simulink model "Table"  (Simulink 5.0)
settings: Solver=FixedStepDiscrete  SolverMode=SingleTasking  StartTime=0.0  StopTime=inf  FixedStep=samplePeriod  RelTol=1e-3  AbsTol=1e-6
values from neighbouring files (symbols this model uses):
  a0 = zeros(1, nAct)    [initialize.m]    (also in quake.m = 0; rspect.m = 1)
  actParamsX = [bulkModulus	* pressCanon,    [initialize.m]
  actParamsY = [bulkModulus	* pressCanon,    [initialize.m]
  actParamsZ = [bulkModulus	* pressCanon,    [initialize.m]
  azMask = zeros(nAcc, 1)    [initialize.m]
  bal = [[ 1  1  1  1  0  0  0  0  0  0  0  0]    [initialize.m]
  cmap = jet    [initialize.m]    (also in tableAnimation.m = self.cmap)
  ea_t = zeros(3, nAcc)    [initialize.m]
  faces = nAct               			+ [ 1  2  3  4    [initialize.m]    (also in tableAnimation.m = self.faces)
  flowCanon = 63090.2    [initialize.m]
  fmax = zeros(nAct, 1)    [initialize.m]
  gasConstant = 1.8    [initialize.m]
  gee = 1.0    (= 1)    [initialize.m]    (also in accelA2T.m = h(24); accelT2A.m = h(24); Test.m)
  inertia = [Ixx 0 0; 0 Iyy 0; 0 0 Izz]    [initialize.m]
  inertiaCanon = 0.1130    (= 0.113)    [initialize.m]
  linAccelCanon = 9800.0    (= 9800)    [initialize.m]    (also in accelA2T.m = h(19); accelT2A.m = h(19); Test.m)
  lines = nAct               			+ [ 1  2  3  4  1    				5  6  7  8  5    				9 10 11 12  9    				0  2  6 10       				0  3  7 11       				0  4  8 12  0];  	lines(find(lines==nAct)) = 0    [initialize.m]    (also in tableAnimation.m = self.lines; viewer.m = 1)
  linVelocCanon = 1000.0    (= 1000)    [initialize.m]    (also in Test.m)
  mass = [massX massY massZ]'    [initialize.m]
  massCanon = 0.4535924e-06    (= 4.535924e-07)    [initialize.m]
  maxDispl = [maxDisplX  			maxDisplY  			maxDisplZ  			maxDisplZ * linVelocCanon / rollRadius  * 180/pi  			maxDisplZ * linVelocCanon / pitchRadius * 180/pi  			min(maxDisplX, maxDisplY) * linVelocCanon / yawRadius * 180/pi]    [initialize.m]
  maxOilVolume = volume * (1 - (precharge/supplyPress)^(1/gasConstant))    (= 32.2704137442)    [initialize.m]
  maxVeloc = [maxVelocX  			maxVelocY  			maxVelocZ  			maxVelocZ * linVelocCanon / rollRadius  * 180/pi  			maxVelocZ * linVelocCanon / pitchRadius * 180/pi  			min(maxVelocX, maxVelocY) * linVelocCanon / yawRadius * 180/pi]    [initialize.m]
  minDispl = -maxDispl    [initialize.m]
  minVeloc = -maxVeloc    [initialize.m]
  nAct = size(rt_t, 2)    [initialize.m]    (also in tableAnimation.m = self.nAct)
  precharge = 2000    [initialize.m]
  pumpFlow = 1e10    (= 10000000000)    [initialize.m]
  ra_t = [  -20.0   -20.0   -92.0 -2590.0  2590.0   -62.0 -2133.0 -2133.0  2133.0  2133.0   -62.0    [initialize.m]    (also in accelA2T.m = [-h9   -h9 -h15 -h10  h10 -h14 -h12 -h12  h12  h12 -h16; accelT2A.m = [-h9   -h9 -h15 -h10  h10 -h14 -h12 -h12  h12  h12 -h16)
  rb_w = [-5692.1 -5692.1  5692.1  5692.1 -2500.0 -2500.0  2500.0  2500.0 -2400.0 -2400.0  2400.0  2400.0    [initialize.m]    (also in tableAnimation.m = rtxrb_w(:,end-nAct+1:end); positT2A.m = [-h4 -h4  h4  h4 -h1 -h1  h1  h1 -h6 -h6  h6  h6)
  returnPress = 50    [initialize.m]
  rgt = -rtg    [initialize.m]
  rotAccelCanon = 1    [initialize.m]    (also in accelA2T.m = h(22); accelT2A.m = h(22); Test.m)
  rotForceCanon = 1000    [initialize.m]    (also in forceA2T.m = h(23); Test.m)
  rotVelocCanon = 1    [initialize.m]    (also in accelA2T.m = h(21); accelT2A.m = h(21); Test.m)
  rt_t = [-3106.4 -3106.4  3106.4  3106.4 -2500.0 -2500.0  2500.0  2500.0 -2400.0 -2400.0  2400.0  2400.0    [initialize.m]    (also in positT2A.m = [rt_tx rt_ty rt_tz])
  rtg = cg    [initialize.m]
  rtx_t = [rt_t	topPlane.topLeft(:)  topPlane.topRight(:)  					topPlane.botRight(:) topPlane.botLeft(:)   					midPlane.topLeft(:)  midPlane.topRight(:)  					midPlane.botRight(:) midPlane.botLeft(:)   					botPlane.topLeft(:)  botPlane.topRight(:)  					botPlane.botRight(:) botPlane.botLeft(:)]    [initialize.m]
  samplePeriod = 1/1024    (= 0.0009765625)    [initialize.m]    (also in viewer.m = eval(getHeaderValue(header, 'DELTA_T')))
  supplyPress = 3000    [initialize.m]
  volume = 160    [initialize.m]    (also in quake.m = volume / 231.0)
  volumeCanon = 3785412.0    (= 3785412)    [initialize.m]
  zlim = [min(rb_w(3,:)) 2*halfLengthZ*lengthCanon]    [initialize.m]
undefined symbols (not defined in the file or in its folder): magnitude
libraries: aerospace x51, simulink x22, simulink_extras x1
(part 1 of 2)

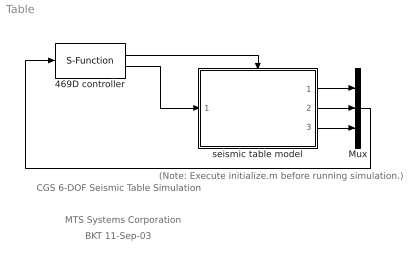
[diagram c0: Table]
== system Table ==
  note: BKT 11-Sep-03
  note: MTS Systems Corporation
  note: CGS 6-DOF Seismic Table Simulation
  note: (Note: Execute initialize.m before running simulation.)
  469D controller : S-Function  FunctionName=mtsConnect  Parameters='127.0.0.1',5002,nAct+nAct+nAcc,nAct
  Mux : Mux  Inputs=3
  seismic table model : Subsystem  TreatAsAtomicUnit=on
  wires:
  seismic table model/1(displ) -> Mux/1
  seismic table model/2(force) -> Mux/2
  seismic table model/3(accel) -> Mux/3
  Mux/1 -> 469D controller/1
  469D controller/1 -> seismic table model/Trigger
  469D controller/2 -> seismic table model/1(valve cmd)

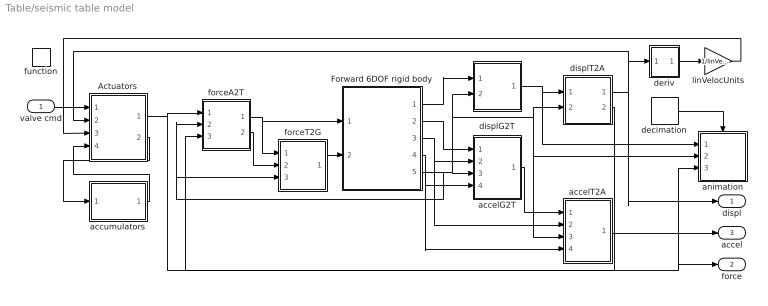
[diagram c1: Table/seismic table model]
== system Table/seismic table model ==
  valve cmd : Inport
  function : TriggerPort  TriggerType=function-call
  Actuators : Subsystem
  Forward 6DOF rigid body : Subsystem
  accelG2T : Subsystem
  accelT2A : Subsystem
  accumulators : Subsystem
  animation : Subsystem  TreatAsAtomicUnit=on  mask{type=2, azim=-37.5, elev=15}
      mask prompts: type "Drawing type (0: none, 1: wire frame, 2: solid)"; azim "View azimuth (degrees)"; elev "View elevation (degrees)"
  decimation : DiscretePulseGenerator  Period=64  SampleTime=-1
  deriv : Subsystem  mask{T=samplePeriod}
      mask prompts: T "Sample period (sec)"
  displG2T : Subsystem
  displT2A : Subsystem
  forceA2T : Subsystem
  forceT2G : Subsystem
  linVelocUnits : Gain  Gain=1/linVelocCanon
  displ : Outport
  force : Outport  Port=2
  accel : Outport  Port=3
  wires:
  valve cmd/1 -> Actuators/1(cmds)
  displT2A/1(out) -> Actuators/2(displ), deriv/1(inp), displ/1
  deriv/1(out) -> linVelocUnits/1
  displT2A/2(dir) -> forceA2T/3(dir)
  Actuators/1(force) -> forceA2T/1(inp), force/1, animation/3(Fact)
  forceA2T/1(xyz) -> forceT2G/1(xyz), Forward 6DOF rigid body/1(Fxyz)
  displG2T/1(out) -> animation/1(xyz), displT2A/1(xyz)
  Forward 6DOF rigid body/5(DCM) -> accelT2A/3(DCM), animation/2(DCM), displT2A/2(DCM), displG2T/2(DCM), accelG2T/3(DCM), forceA2T/2(DCM), forceT2G/3(DCM)
  accelG2T/1(out) -> accelT2A/1(xyz)
  forceA2T/2(rpw) -> forceT2G/2(rpw)
  forceT2G/1(out) -> Forward 6DOF rigid body/2(Mxyz)
  Forward 6DOF rigid body/1(xyz) -> displG2T/1(xyz)
  Forward 6DOF rigid body/4(rot veloc) -> accelT2A/4(rot veloc), accelG2T/4(rot veloc)
  Forward 6DOF rigid body/3(rot accel) -> accelT2A/2(rpw), accelG2T/2(rpw)
  Forward 6DOF rigid body/2(lin accel) -> accelG2T/1(xyz)
  linVelocUnits/1 -> Actuators/3(veloc)
  Actuators/2(flow) -> accumulators/1(flow)
  accumulators/1(press) -> Actuators/4(press)
  accelT2A/1(out) -> accel/1
  decimation/1 -> animation/Trigger

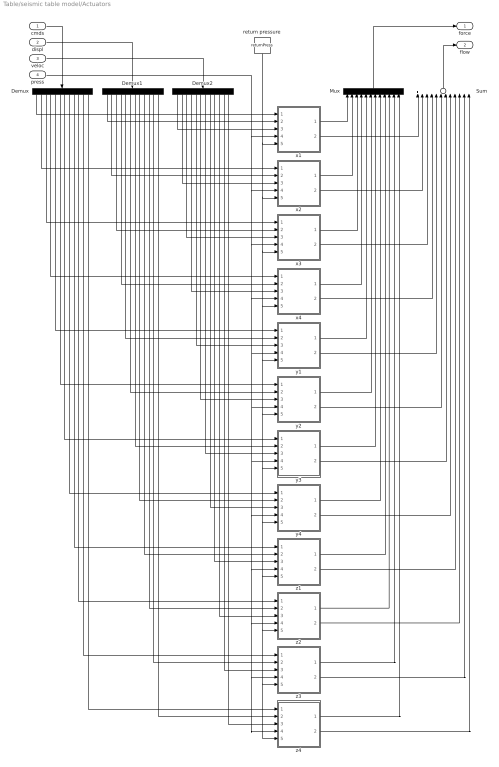
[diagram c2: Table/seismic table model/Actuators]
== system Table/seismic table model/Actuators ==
  cmds : Inport
  displ : Inport  Port=2
  veloc : Inport  Port=3
  press : Inport  Port=4
  Demux : Demux  Orientation=down  Outputs=12
  Demux1 : Demux  Orientation=down  Outputs=12
  Demux2 : Demux  Orientation=down  Outputs=12
  Mux : Mux  Orientation=up  Inputs=12
  Sum : Sum  Orientation=up  Inputs=12
  return pressure : Constant  Orientation=down  Value=returnPress
  x1 : Subsystem  mask(Inverse Actuator){params=actParamsX}
      mask prompts: params "Parameter vector"
  x2 : Subsystem  mask(Inverse Actuator){params=actParamsX}
      mask prompts: params "Parameter vector"
  x3 : Subsystem  mask(Inverse Actuator){params=actParamsX}
      mask prompts: params "Parameter vector"
  x4 : Subsystem  mask(Inverse Actuator){params=actParamsX}
      mask prompts: params "Parameter vector"
  y1 : Subsystem  mask(Inverse Actuator){params=actParamsY}
      mask prompts: params "Parameter vector"
  y2 : Subsystem  mask(Inverse Actuator){params=actParamsY}
      mask prompts: params "Parameter vector"
  y3 : Subsystem  mask(Inverse Actuator){params=actParamsY}
      mask prompts: params "Parameter vector"
  y4 : Subsystem  mask(Inverse Actuator){params=actParamsY}
      mask prompts: params "Parameter vector"
  z1 : Subsystem  mask(Inverse Actuator){params=actParamsZ}
      mask prompts: params "Parameter vector"
  z2 : Subsystem  mask(Inverse Actuator){params=actParamsZ}
      mask prompts: params "Parameter vector"
  z3 : Subsystem  mask(Inverse Actuator){params=actParamsZ}
      mask prompts: params "Parameter vector"
  z4 : Subsystem  mask(Inverse Actuator){params=actParamsZ}
      mask prompts: params "Parameter vector"
  force : Outport
  flow : Outport  Port=2
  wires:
  cmds/1 -> Demux/1
  displ/1 -> Demux1/1
  Demux/1 -> x1/1(cmd)
  Demux/2 -> x2/1(cmd)
  Demux1/1 -> x1/2(displ)
  Demux2/1 -> x1/3(veloc)
  Demux1/2 -> x2/2(displ)
  Demux2/2 -> x2/3(veloc)
  Demux/3 -> x3/1(cmd)
  Demux1/3 -> x3/2(displ)
  Demux2/3 -> x3/3(veloc)
  Demux/4 -> x4/1(cmd)
  Demux1/4 -> x4/2(displ)
  Demux2/4 -> x4/3(veloc)
  Demux/5 -> y1/1(cmd)
  Demux1/5 -> y1/2(displ)
  Demux2/5 -> y1/3(veloc)
  Demux/6 -> y2/1(cmd)
  Demux1/6 -> y2/2(displ)
  Demux2/6 -> y2/3(veloc)
  Demux/7 -> y3/1(cmd)
  Demux1/7 -> y3/2(displ)
  Demux2/7 -> y3/3(veloc)
  Demux/8 -> y4/1(cmd)
  Demux1/8 -> y4/2(displ)
  Demux2/8 -> y4/3(veloc)
  x1/1(force) -> Mux/1
  x2/1(force) -> Mux/2
  x3/1(force) -> Mux/3
  x4/1(force) -> Mux/4
  Mux/1 -> force/1
  y1/1(force) -> Mux/5
  y2/1(force) -> Mux/6
  y3/1(force) -> Mux/7
  y4/1(force) -> Mux/8
  veloc/1 -> Demux2/1
  press/1 -> z3/4(spl press), z4/4(spl press), z2/4(spl press), z1/4(spl press), y4/4(spl press), y3/4(spl press), y2/4(spl press), y1/4(spl press), x4/4(spl press), x3/4(spl press), x2/4(spl press), x1/4(spl press)
  return pressure/1 -> z3/5(rtn press), z4/5(rtn press), z2/5(rtn press), z1/5(rtn press), y4/5(rtn press), y3/5(rtn press), y2/5(rtn press), y1/5(rtn press), x4/5(rtn press), x3/5(rtn press), x2/5(rtn press), x1/5(rtn press)
  Sum/1 -> flow/1
  x1/2(flow) -> Sum/1
  x2/2(flow) -> Sum/2
  x3/2(flow) -> Sum/3
  x4/2(flow) -> Sum/4
  y1/2(flow) -> Sum/5
  y2/2(flow) -> Sum/6
  y3/2(flow) -> Sum/7
  y4/2(flow) -> Sum/8
  Demux/9 -> z1/1(cmd)
  Demux/11 -> z3/1(cmd)
  Demux/10 -> z2/1(cmd)
  Demux/12 -> z4/1(cmd)
  Demux1/9 -> z1/2(displ)
  Demux1/10 -> z2/2(displ)
  Demux1/11 -> z3/2(displ)
  Demux1/12 -> z4/2(displ)
  Demux2/9 -> z1/3(veloc)
  Demux2/10 -> z2/3(veloc)
  Demux2/11 -> z3/3(veloc)
  Demux2/12 -> z4/3(veloc)
  z1/1(force) -> Mux/9
  z2/1(force) -> Mux/10
  z3/1(force) -> Mux/11
  z4/1(force) -> Mux/12
  z1/2(flow) -> Sum/9
  z2/2(flow) -> Sum/10
  z3/2(flow) -> Sum/11
  z4/2(flow) -> Sum/12

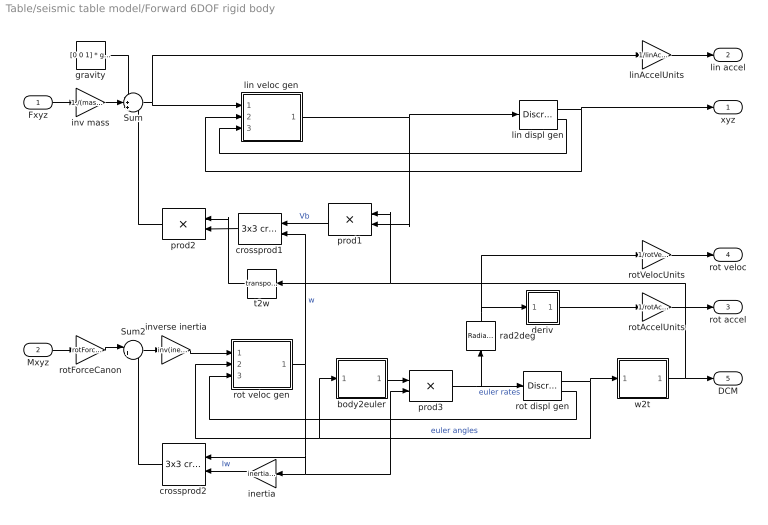
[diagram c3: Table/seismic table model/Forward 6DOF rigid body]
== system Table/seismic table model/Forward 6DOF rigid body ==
  Fxyz : Inport
  Mxyz : Inport  Port=2
  Sum : Sum  Inputs=-++
  Sum2 : Sum  Inputs=|+-
  body2euler : Subsystem
  crossprod1 : aerospace/Axes Transformations/3x3 cross product  Orientation=left
  crossprod2 : aerospace/Axes Transformations/3x3 cross product  Orientation=left
  deriv : Subsystem  mask{T=samplePeriod}
      mask prompts: T "Sample period (sec)"
  gravity : Constant  Value=[0 0 1] * gee * linAccelCanon * ~static
  inertia : Gain  Orientation=left  Gain=inertia*inertiaCanon  Multiplication=Matrix(K*u)
  inv mass : Gain  Gain=1./(mass*massCanon)
  inverse inertia : Gain  Gain=inv(inertia*inertiaCanon)  Multiplication=Matrix(K*u)
  lin displ gen : DiscreteIntegrator  IntegratorMethod=Backward Euler  LimitOutput=on  UpperSaturationLimit=maxDispl(1:3)  LowerSaturationLimit=minDispl(1:3)  ShowSaturationPort=on  SampleTime=-1
  lin veloc gen : Subsystem  mask{maxVeloc=maxVeloc(1:3)*linVelocCanon, minVeloc=minVeloc(1:3)*linVelocCanon, maxDispl=maxDispl(1:3), minDispl=minDispl(1:3)}
      mask prompts: maxVeloc "Max velocity"; minVeloc "Min velocity"; maxDispl "Max displacement"; minDispl "Min displacement"
  linAccelUnits : Gain  Gain=1/linAccelCanon
  prod1 : Product  Orientation=left  Multiplication=Matrix(*)
  prod2 : Product  Orientation=left  Multiplication=Matrix(*)
  prod3 : Product  Multiplication=Matrix(*)
  rad2deg : simulink_extras/Transformations/Radians to Degrees  Orientation=up
  rot displ gen : DiscreteIntegrator  LimitOutput=on  UpperSaturationLimit=maxDispl(4:6)*pi/180  LowerSaturationLimit=minDispl(4:6)*pi/180  ShowSaturationPort=on  SampleTime=-1
  rot veloc gen : Subsystem  mask{maxVeloc=maxVeloc(4:6)*rotVelocCanon*pi/180, minVeloc=minVeloc(4:6)*rotVelocCanon*pi/180, maxDispl=maxDispl(4:6)*pi/180, minDispl=minDispl(4:6)*pi/180}
      mask prompts: maxVeloc "Max velocity"; minVeloc "Min velocity"; maxDispl "Max displacement"; minDispl "Min displacement"
  rotAccelUnits : Gain  Gain=1/rotAccelCanon
  rotForceCanon : Gain  Gain=rotForceCanon
  rotVelocUnits : Gain  Gain=1/rotVelocCanon
  t2w : Math  Orientation=left  Operator=transpose
  w2t : Subsystem
  xyz : Outport
  lin accel : Outport  Port=2
  rot accel : Outport  Port=3
  rot veloc : Outport  Port=4
  DCM : Outport  Port=5
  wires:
  inertia/1 -> crossprod2/2  "Iw"
  Sum2/1 -> inverse inertia/1
  rot veloc gen/1(veloc) -> crossprod1/2, crossprod2/1, inertia/1, prod3/2  "w"
  lin veloc gen/1(veloc) -> prod1/2, lin displ gen/1
  Mxyz/1 -> rotForceCanon/1
  body2euler/1(out) -> prod3/1
  prod3/1 -> rad2deg/1, rot displ gen/1  "euler rates"
  w2t/1(DCM) -> t2w/1, prod1/1, DCM/1
  rotVelocUnits/1 -> rot veloc/1
  rotForceCanon/1 -> Sum2/1
  linAccelUnits/1 -> lin accel/1
  lin displ gen/1 -> xyz/1, lin veloc gen/2(displ)
  gravity/1 -> Sum/1
  Fxyz/1 -> inv mass/1
  inv mass/1 -> Sum/2
  Sum/1 -> linAccelUnits/1, lin veloc gen/1(accel)
  crossprod1/1 -> prod2/2
  prod2/1 -> Sum/3
  t2w/1 -> prod2/1
  prod1/1 -> crossprod1/1  "Vb"
  rotAccelUnits/1 -> rot accel/1
  rot displ gen/1 -> w2t/1(rpw), body2euler/1(rpw), rot veloc gen/2(displ)  "euler angles"
  deriv/1(out) -> rotAccelUnits/1
  crossprod2/1 -> Sum2/2
  rad2deg/1 -> deriv/1(inp), rotVelocUnits/1
  lin displ gen/2 -> lin veloc gen/3(reset)
  inverse inertia/1 -> rot veloc gen/1(accel)
  rot displ gen/2 -> rot veloc gen/3(reset)

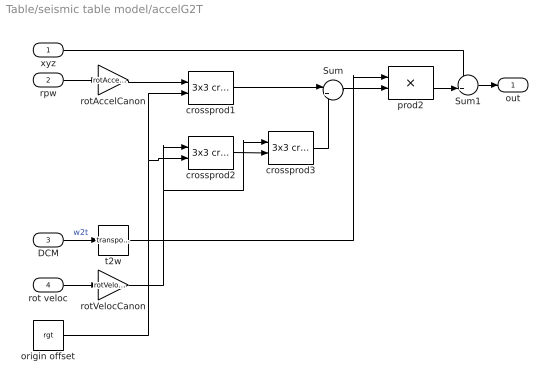
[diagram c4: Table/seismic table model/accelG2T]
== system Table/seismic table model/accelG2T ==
  xyz : Inport
  rpw : Inport  Port=2
  DCM : Inport  Port=3
  rot veloc : Inport  Port=4
  Sum : Sum  Inputs=|++
  Sum1 : Sum  Inputs=++|
  crossprod1 : aerospace/Axes Transformations/3x3 cross product
  crossprod2 : aerospace/Axes Transformations/3x3 cross product
  crossprod3 : aerospace/Axes Transformations/3x3 cross product
  origin offset : Constant  Value=rgt
  prod2 : Product  Multiplication=Matrix(*)
  rotAccelCanon : Gain  Gain=rotAccelCanon*(pi/180)/linAccelCanon
  rotVelocCanon : Gain  Gain=rotVelocCanon*(pi/180)/sqrt(linAccelCanon)
  t2w : Math  Operator=transpose
  out : Outport
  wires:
  rotVelocCanon/1 -> crossprod2/1, crossprod3/1
  DCM/1 -> t2w/1  "w2t"
  rot veloc/1 -> rotVelocCanon/1
  xyz/1 -> Sum1/1
  t2w/1 -> prod2/1
  rpw/1 -> rotAccelCanon/1
  rotAccelCanon/1 -> crossprod1/1
  origin offset/1 -> crossprod2/2, crossprod1/2
  Sum/1 -> prod2/2
  crossprod2/1 -> crossprod3/2
  prod2/1 -> Sum1/2
  Sum1/1 -> out/1
  crossprod3/1 -> Sum/2
  crossprod1/1 -> Sum/1

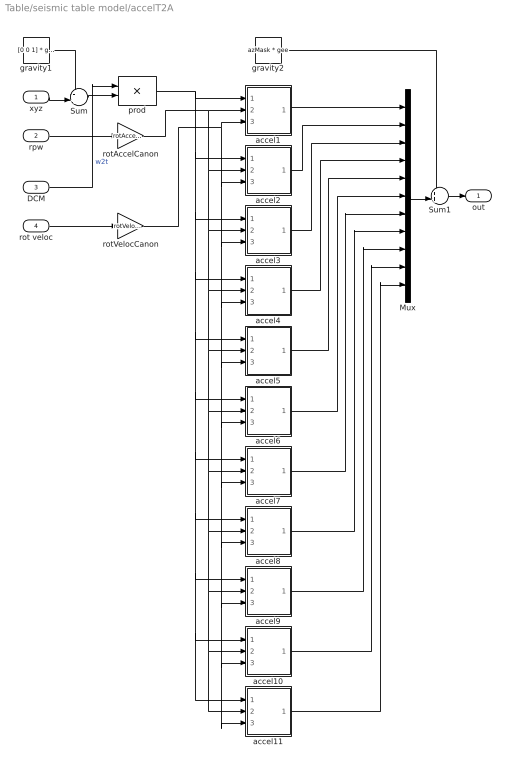
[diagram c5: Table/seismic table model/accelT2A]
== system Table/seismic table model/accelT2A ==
  xyz : Inport
  rpw : Inport  Port=2
  DCM : Inport  Port=3
  rot veloc : Inport  Port=4
  Mux : Mux  Inputs=11
  Sum : Sum  Inputs=-+|
  Sum1 : Sum  Inputs=++|
  accel1 : Subsystem  mask{id=1}
      mask prompts: id "Accelerometer number"
  accel10 : Subsystem  mask{id=10}
      mask prompts: id "Accelerometer number"
  accel11 : Subsystem  mask{id=11}
      mask prompts: id "Accelerometer number"
  accel2 : Subsystem  mask{id=2}
      mask prompts: id "Accelerometer number"
  accel3 : Subsystem  mask{id=3}
      mask prompts: id "Accelerometer number"
  accel4 : Subsystem  mask{id=4}
      mask prompts: id "Accelerometer number"
  accel5 : Subsystem  mask{id=5}
      mask prompts: id "Accelerometer number"
  accel6 : Subsystem  mask{id=6}
      mask prompts: id "Accelerometer number"
  accel7 : Subsystem  mask{id=7}
      mask prompts: id "Accelerometer number"
  accel8 : Subsystem  mask{id=8}
      mask prompts: id "Accelerometer number"
  accel9 : Subsystem  mask{id=9}
      mask prompts: id "Accelerometer number"
  gravity1 : Constant  Value=[0 0 1] * gee
  gravity2 : Constant  Value=azMask * gee
  prod : Product  Multiplication=Matrix(*)
  rotAccelCanon : Gain  Gain=rotAccelCanon*(pi/180)/linAccelCanon
  rotVelocCanon : Gain  Gain=rotVelocCanon*(pi/180)/sqrt(linAccelCanon)
  out : Outport
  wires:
  prod/1 -> accel10/1(linacc), accel11/1(linacc), accel9/1(linacc), accel8/1(linacc), accel7/1(linacc), accel6/1(linacc), accel5/1(linacc), accel4/1(linacc), accel3/1(linacc), accel2/1(linacc), accel1/1(linacc)
  rpw/1 -> rotAccelCanon/1
  rot veloc/1 -> rotVelocCanon/1
  DCM/1 -> prod/1  "w2t"
  rotVelocCanon/1 -> accel10/3(rotvel), accel11/3(rotvel), accel9/3(rotvel), accel8/3(rotvel), accel7/3(rotvel), accel6/3(rotvel), accel5/3(rotvel), accel4/3(rotvel), accel3/3(rotvel), accel2/3(rotvel), accel1/3(rotvel)
  rotAccelCanon/1 -> accel10/2(rotacc), accel11/2(rotacc), accel9/2(rotacc), accel8/2(rotacc), accel7/2(rotacc), accel6/2(rotacc), accel5/2(rotacc), accel4/2(rotacc), accel3/2(rotacc), accel2/2(rotacc), accel1/2(rotacc)
  accel1/1(out) -> Mux/1
  accel2/1(out) -> Mux/2
  accel6/1(out) -> Mux/6
  accel5/1(out) -> Mux/5
  accel4/1(out) -> Mux/4
  accel3/1(out) -> Mux/3
  Sum/1 -> prod/2
  xyz/1 -> Sum/2
  gravity1/1 -> Sum/1
  accel11/1(out) -> Mux/11
  accel10/1(out) -> Mux/10
  accel9/1(out) -> Mux/9
  accel8/1(out) -> Mux/8
  accel7/1(out) -> Mux/7
  Mux/1 -> Sum1/2
  Sum1/1 -> out/1
  gravity2/1 -> Sum1/1

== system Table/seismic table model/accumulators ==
  flow : Inport
  Sum : Sum  Inputs=+-|
  Sum1 : Sum  Inputs=+-|
  bottle volume : Constant  Value=volume*volumeCanon
  flowCanon : Gain  Gain=flowCanon
  gas constant : Constant  Value=gasConstant
  initial condition : UnitDelay  X0=supplyPress  SampleTime=-1
  integrator : DiscreteIntegrator  InitialCondition=maxOilVolume*volumeCanon  LimitOutput=on  UpperSaturationLimit=maxOilVolume*volumeCanon  LowerSaturationLimit=0  SampleTime=-1
  power : Math  Operator=pow
  precharge : Gain  Gain=precharge
  pump flow : Constant  Value=pumpFlow
  quotient : Product  Inputs=*/
  press : Outport
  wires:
  pump flow/1 -> Sum/1
  Sum/1 -> flowCanon/1
  bottle volume/1 -> Sum1/1, quotient/1
  gas constant/1 -> power/2
  power/1 -> precharge/1
  precharge/1 -> initial condition/1
  Sum1/1 -> quotient/2  "current gas volume"
  quotient/1 -> power/1
  integrator/1 -> Sum1/2  "current oil volume"
  flow/1 -> Sum/2
  flowCanon/1 -> integrator/1
  initial condition/1 -> press/1

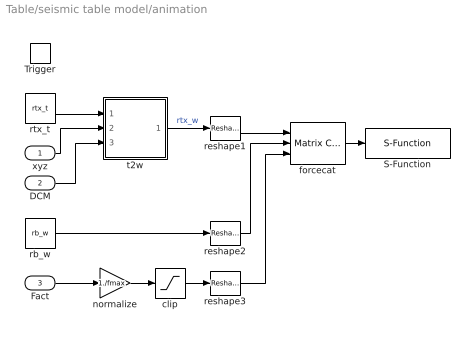
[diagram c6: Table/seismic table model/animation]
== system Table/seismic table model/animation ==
  xyz : Inport
  DCM : Inport  Port=2
  Fact : Inport  Port=3
  Trigger : TriggerPort
  S-Function : S-Function  FunctionName=tableAnimation  Parameters=type,azim,elev,nAct,zlim,lines,faces,cmap
  clip : Saturate  UpperLimit=1  LowerLimit=-1
  forcecat : simulink/Math Operations/Matrix Concatenation  numInports=3  catMethod=Vertical
  normalize : Gain  Gain=1./fmax
  rb_w : Constant  Value=rb_w
  reshape1 : simulink/Math Operations/Reshape  OutputDimensionality=1-D array  OutputDimensions=[1,1]
  reshape2 : simulink/Math Operations/Reshape  OutputDimensionality=1-D array  OutputDimensions=[1,1]
  reshape3 : simulink/Math Operations/Reshape  OutputDimensionality=1-D array  OutputDimensions=[1,1]
  rtx_t : Constant  Value=rtx_t
  t2w : Subsystem
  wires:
  DCM/1 -> t2w/3(DCM)
  xyz/1 -> t2w/2(xyz)
  rtx_t/1 -> t2w/1(inp)
  reshape3/1 -> forcecat/3
  reshape2/1 -> forcecat/2
  rb_w/1 -> reshape2/1
  forcecat/1 -> S-Function/1
  reshape1/1 -> forcecat/1
  Fact/1 -> normalize/1
  t2w/1(out) -> reshape1/1  "rtx_w"
  normalize/1 -> clip/1
  clip/1 -> reshape3/1

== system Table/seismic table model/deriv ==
  inp : Inport
  1/T : Gain  Gain=1/T
  Sum : Sum  Inputs=|+-
  Unit Delay : UnitDelay  SampleTime=-1
  out : Outport
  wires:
  1/T/1 -> out/1
  Sum/1 -> 1/T/1
  Unit Delay/1 -> Sum/2
  inp/1 -> Unit Delay/1, Sum/1

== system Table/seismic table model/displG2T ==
  xyz : Inport
  DCM : Inport  Port=2
  Sum1 : Sum  Inputs=++-
  origin offset : Constant  Value=rgt
  prod : Product  Multiplication=Matrix(*)
  t2w : Math  Operator=transpose
  out : Outport
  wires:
  t2w/1 -> prod/1
  DCM/1 -> t2w/1
  origin offset/1 -> prod/2, Sum1/3
  xyz/1 -> Sum1/1
  prod/1 -> Sum1/2
  Sum1/1 -> out/1

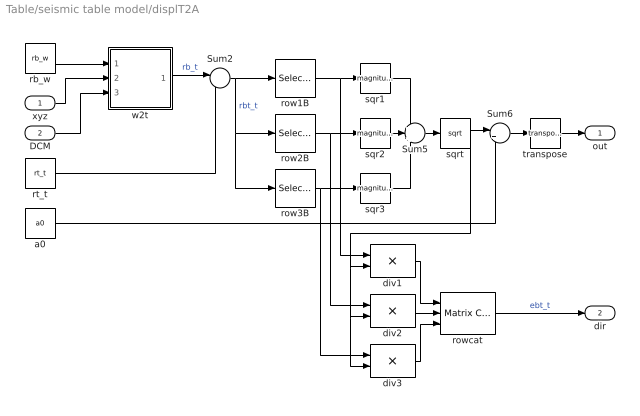
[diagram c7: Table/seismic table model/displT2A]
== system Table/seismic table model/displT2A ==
  xyz : Inport
  DCM : Inport  Port=2
  Sum2 : Sum  Inputs=|-+
  Sum5 : Sum  Inputs=+++
  Sum6 : Sum  Inputs=|+-
  a0 : Constant  Value=a0
  div1 : Product  Inputs=*/
  div2 : Product  Inputs=*/
  div3 : Product  Inputs=*/
  rb_w : Constant  Value=rb_w
  row1B : Selector  InputType=Matrix  Elements=[1 3]  Columns=-1  InputPortWidth=3
  row2B : Selector  InputType=Matrix  Elements=[1 3]  Rows=2  Columns=-1  InputPortWidth=3
  row3B : Selector  InputType=Matrix  Elements=[1 3]  Rows=3  Columns=-1  InputPortWidth=3
  rowcat : simulink/Math Operations/Matrix Concatenation  numInports=3  catMethod=Vertical
  rt_t : Constant  Value=rt_t
  sqr1 : Math  Operator=magnitude^2
  sqr2 : Math  Operator=magnitude^2
  sqr3 : Math  Operator=magnitude^2
  sqrt : Math  Operator=sqrt
  transpose : Math  Operator=transpose
  w2t : Subsystem
  out : Outport
  dir : Outport  Port=2
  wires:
  xyz/1 -> w2t/2(xyz)
  rb_w/1 -> w2t/1(inp)
  rt_t/1 -> Sum2/2
  row2B/1 -> sqr2/1, div2/1
  row1B/1 -> sqr1/1, div1/1
  row3B/1 -> sqr3/1, div3/1
  Sum5/1 -> sqrt/1
  a0/1 -> Sum6/2
  sqrt/1 -> Sum6/1, div1/2, div2/2, div3/2
  w2t/1(out) -> Sum2/1  "rb_t"
  Sum2/1 -> row3B/1, row2B/1, row1B/1  "rbt_t"
  sqr1/1 -> Sum5/1
  sqr2/1 -> Sum5/2
  sqr3/1 -> Sum5/3
  rowcat/1 -> dir/1  "ebt_t"
  div1/1 -> rowcat/1
  div2/1 -> rowcat/2
  div3/1 -> rowcat/3
  DCM/1 -> w2t/3(DCM)
  Sum6/1 -> transpose/1
  transpose/1 -> out/1

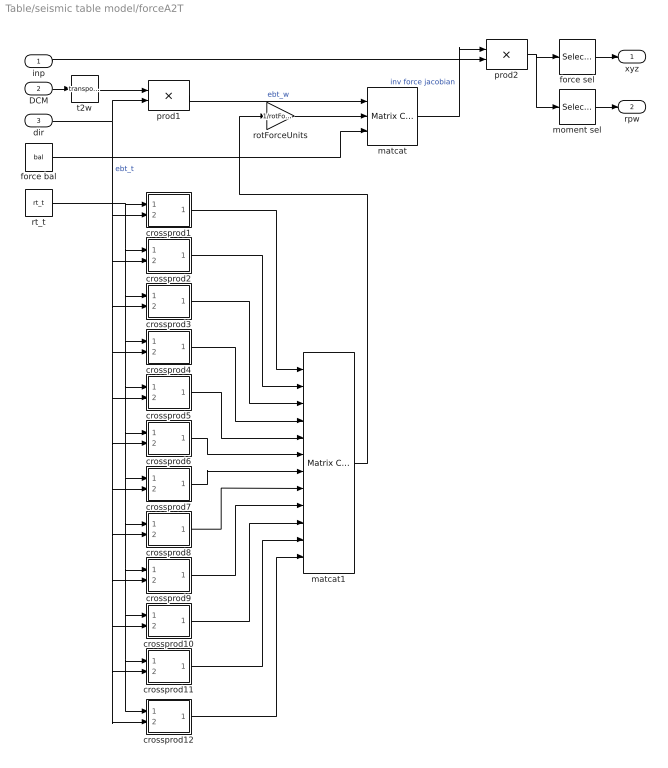
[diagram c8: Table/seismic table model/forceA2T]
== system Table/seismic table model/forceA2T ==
  inp : Inport
  DCM : Inport  Port=2
  dir : Inport  Port=3
  crossprod1 : Subsystem  mask{id=1}
      mask prompts: id "Actuator number"
  crossprod10 : Subsystem  mask{id=10}
      mask prompts: id "Actuator number"
  crossprod11 : Subsystem  mask{id=11}
      mask prompts: id "Actuator number"
  crossprod12 : Subsystem  mask{id=12}
      mask prompts: id "Actuator number"
  crossprod2 : Subsystem  mask{id=2}
      mask prompts: id "Actuator number"
  crossprod3 : Subsystem  mask{id=3}
      mask prompts: id "Actuator number"
  crossprod4 : Subsystem  mask{id=4}
      mask prompts: id "Actuator number"
  crossprod5 : Subsystem  mask{id=5}
      mask prompts: id "Actuator number"
  crossprod6 : Subsystem  mask{id=6}
      mask prompts: id "Actuator number"
  crossprod7 : Subsystem  mask{id=7}
      mask prompts: id "Actuator number"
  crossprod8 : Subsystem  mask{id=8}
      mask prompts: id "Actuator number"
  crossprod9 : Subsystem  mask{id=9}
      mask prompts: id "Actuator number"
  force bal : Constant  Value=bal
  force sel : Selector  Elements=[1 2 3]
  matcat : simulink/Math Operations/Matrix Concatenation  numInports=3  catMethod=Vertical
  matcat1 : simulink/Math Operations/Matrix Concatenation  numInports=12  catMethod=Horizontal
  moment sel : Selector  Elements=[4 5 6]
  prod1 : Product  Multiplication=Matrix(*)
  prod2 : Product  Multiplication=Matrix(*)
  rotForceUnits : Gain  Gain=1/rotForceCanon
  rt_t : Constant  Value=rt_t
  t2w : Math  Operator=transpose
  xyz : Outport
  rpw : Outport  Port=2
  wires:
  rotForceUnits/1 -> matcat/2
  matcat/1 -> prod2/1  "inv force jacobian"
  force sel/1 -> xyz/1
  moment sel/1 -> rpw/1
  DCM/1 -> t2w/1
  dir/1 -> prod1/2, crossprod1/2(B), crossprod7/2(B), crossprod8/2(B), crossprod12/2(B), crossprod11/2(B), crossprod10/2(B), crossprod9/2(B), crossprod6/2(B), crossprod5/2(B), crossprod4/2(B), crossprod3/2(B), crossprod2/2(B)  "ebt_t"
  prod1/1 -> matcat/1  "ebt_w"
  rt_t/1 -> crossprod1/1(A), crossprod7/1(A), crossprod8/1(A), crossprod12/1(A), crossprod11/1(A), crossprod10/1(A), crossprod9/1(A), crossprod6/1(A), crossprod5/1(A), crossprod4/1(A), crossprod3/1(A), crossprod2/1(A)
  matcat1/1 -> rotForceUnits/1
  crossprod1/1(AxB) -> matcat1/1
  crossprod2/1(AxB) -> matcat1/2
  crossprod3/1(AxB) -> matcat1/3
  crossprod4/1(AxB) -> matcat1/4
  crossprod5/1(AxB) -> matcat1/5
  crossprod6/1(AxB) -> matcat1/6
  crossprod7/1(AxB) -> matcat1/7
  crossprod8/1(AxB) -> matcat1/8
  inp/1 -> prod2/2
  t2w/1 -> prod1/1
  prod2/1 -> force sel/1, moment sel/1
  force bal/1 -> matcat/3
  crossprod12/1(AxB) -> matcat1/12
  crossprod11/1(AxB) -> matcat1/11
  crossprod10/1(AxB) -> matcat1/10
  crossprod9/1(AxB) -> matcat1/9

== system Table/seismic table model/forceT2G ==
  xyz : Inport
  rpw : Inport  Port=2
  DCM : Inport  Port=3
  Sum : Sum  Inputs=++|
  crossprod : aerospace/Axes Transformations/3x3 cross product
  origin offset : Constant  Value=rtg
  prod : Product  Multiplication=Matrix(*)
  rotForceUnits : Gain  Gain=1/rotForceCanon
  out : Outport
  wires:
  rpw/1 -> Sum/2
  Sum/1 -> out/1
  crossprod/1 -> rotForceUnits/1
  rotForceUnits/1 -> Sum/1
  xyz/1 -> prod/2
  DCM/1 -> prod/1
  prod/1 -> crossprod/1
  origin offset/1 -> crossprod/2

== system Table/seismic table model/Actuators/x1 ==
  note: Auxiliary diagnostic output vector: 1: valve opening 2: C1 pressure 3: C2 pressure 4: delta pressure 5: force 6: velocity 7: C1 flow 8: C2 flow 9: total flow 10: kinematic flow 11: compressibility flow 12: leakage flow
  note: Note: "1" and "2" denote actuator cylinders on either side of the actuator piston. With positive valve drive, oil is ported into cylinder 1, resulting in positive displacement.
  note: Parameter vector: 1: oil bulk modulus (force/displ^2) 2: servovalve natural frequency (Hz) 3: servovalve damping ratio 4: servovalve overlap 5: rated pressure (force/displ^2) 6: flow at rated pressure (displ^3/sec) 7: actuator piston area 1 (displ^2) 8: actuator piston area 2 (displ^2) 9: actuator usable stroke 1 (displ) 10: actuator usable stroke 2 (displ) 11: actuator end cushion length 1 (displ) 12: actuator end cushion length 2 (displ) 13: actuator parasitic damping factor 14: cross-chamber leakage factor (flow/press) 15: ratio port openings according to area 16: sample period (sec) Conversion factors used for converting signals from external (user) to internal (canonical) units: 17: displacement 18: velocity 19: force 20: pressure 21: flow
  cmd : Inport
  displ : Inport  Port=2
  veloc : Inport  Port=3
  spl press : Inport  Port=4
  rtn press : Inport  Port=5
  abs : Abs
  actuator : S-Function  FunctionName=actuator  Parameters=params
  total flow sel : Selector  Elements=9  InputPortWidth=12
  force : Outport
  flow : Outport  Port=2
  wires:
  spl press/1 -> actuator/4
  rtn press/1 -> actuator/5
  cmd/1 -> actuator/1
  actuator/1 -> force/1
  displ/1 -> actuator/2
  veloc/1 -> actuator/3
  actuator/2 -> total flow sel/1
  total flow sel/1 -> abs/1
  abs/1 -> flow/1

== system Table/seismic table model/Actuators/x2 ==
  note: Parameter vector: 1: oil bulk modulus (force/displ^2) 2: servovalve natural frequency (Hz) 3: servovalve damping ratio 4: servovalve overlap 5: rated pressure (force/displ^2) 6: flow at rated pressure (displ^3/sec) 7: actuator piston area 1 (displ^2) 8: actuator piston area 2 (displ^2) 9: actuator usable stroke 1 (displ) 10: actuator usable stroke 2 (displ) 11: actuator end cushion length 1 (displ) 12: actuator end cushion length 2 (displ) 13: actuator parasitic damping factor 14: cross-chamber leakage factor (flow/press) 15: ratio port openings according to area 16: sample period (sec) Conversion factors used for converting signals from external (user) to internal (canonical) units: 17: displacement 18: velocity 19: force 20: pressure 21: flow
  note: Note: "1" and "2" denote actuator cylinders on either side of the actuator piston. With positive valve drive, oil is ported into cylinder 1, resulting in positive displacement.
  note: Auxiliary diagnostic output vector: 1: valve opening 2: C1 pressure 3: C2 pressure 4: delta pressure 5: force 6: velocity 7: C1 flow 8: C2 flow 9: total flow 10: kinematic flow 11: compressibility flow 12: leakage flow
  cmd : Inport
  displ : Inport  Port=2
  veloc : Inport  Port=3
  spl press : Inport  Port=4
  rtn press : Inport  Port=5
  abs : Abs
  actuator : S-Function  FunctionName=actuator  Parameters=params
  total flow sel : Selector  Elements=9  InputPortWidth=12
  force : Outport
  flow : Outport  Port=2
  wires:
  abs/1 -> flow/1
  total flow sel/1 -> abs/1
  actuator/2 -> total flow sel/1
  veloc/1 -> actuator/3
  displ/1 -> actuator/2
  actuator/1 -> force/1
  cmd/1 -> actuator/1
  rtn press/1 -> actuator/5
  spl press/1 -> actuator/4

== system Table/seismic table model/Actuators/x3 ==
  note: Auxiliary diagnostic output vector: 1: valve opening 2: C1 pressure 3: C2 pressure 4: delta pressure 5: force 6: velocity 7: C1 flow 8: C2 flow 9: total flow 10: kinematic flow 11: compressibility flow 12: leakage flow
  note: Note: "1" and "2" denote actuator cylinders on either side of the actuator piston. With positive valve drive, oil is ported into cylinder 1, resulting in positive displacement.
  note: Parameter vector: 1: oil bulk modulus (force/displ^2) 2: servovalve natural frequency (Hz) 3: servovalve damping ratio 4: servovalve overlap 5: rated pressure (force/displ^2) 6: flow at rated pressure (displ^3/sec) 7: actuator piston area 1 (displ^2) 8: actuator piston area 2 (displ^2) 9: actuator usable stroke 1 (displ) 10: actuator usable stroke 2 (displ) 11: actuator end cushion length 1 (displ) 12: actuator end cushion length 2 (displ) 13: actuator parasitic damping factor 14: cross-chamber leakage factor (flow/press) 15: ratio port openings according to area 16: sample period (sec) Conversion factors used for converting signals from external (user) to internal (canonical) units: 17: displacement 18: velocity 19: force 20: pressure 21: flow
  cmd : Inport
  displ : Inport  Port=2
  veloc : Inport  Port=3
  spl press : Inport  Port=4
  rtn press : Inport  Port=5
  abs : Abs
  actuator : S-Function  FunctionName=actuator  Parameters=params
  total flow sel : Selector  Elements=9  InputPortWidth=12
  force : Outport
  flow : Outport  Port=2
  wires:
  spl press/1 -> actuator/4
  rtn press/1 -> actuator/5
  cmd/1 -> actuator/1
  actuator/1 -> force/1
  displ/1 -> actuator/2
  veloc/1 -> actuator/3
  actuator/2 -> total flow sel/1
  total flow sel/1 -> abs/1
  abs/1 -> flow/1

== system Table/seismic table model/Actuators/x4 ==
  note: Parameter vector: 1: oil bulk modulus (force/displ^2) 2: servovalve natural frequency (Hz) 3: servovalve damping ratio 4: servovalve overlap 5: rated pressure (force/displ^2) 6: flow at rated pressure (displ^3/sec) 7: actuator piston area 1 (displ^2) 8: actuator piston area 2 (displ^2) 9: actuator usable stroke 1 (displ) 10: actuator usable stroke 2 (displ) 11: actuator end cushion length 1 (displ) 12: actuator end cushion length 2 (displ) 13: actuator parasitic damping factor 14: cross-chamber leakage factor (flow/press) 15: ratio port openings according to area 16: sample period (sec) Conversion factors used for converting signals from external (user) to internal (canonical) units: 17: displacement 18: velocity 19: force 20: pressure 21: flow
  note: Note: "1" and "2" denote actuator cylinders on either side of the actuator piston. With positive valve drive, oil is ported into cylinder 1, resulting in positive displacement.
  note: Auxiliary diagnostic output vector: 1: valve opening 2: C1 pressure 3: C2 pressure 4: delta pressure 5: force 6: velocity 7: C1 flow 8: C2 flow 9: total flow 10: kinematic flow 11: compressibility flow 12: leakage flow
  cmd : Inport
  displ : Inport  Port=2
  veloc : Inport  Port=3
  spl press : Inport  Port=4
  rtn press : Inport  Port=5
  abs : Abs
  actuator : S-Function  FunctionName=actuator  Parameters=params
  total flow sel : Selector  Elements=9  InputPortWidth=12
  force : Outport
  flow : Outport  Port=2
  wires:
  abs/1 -> flow/1
  total flow sel/1 -> abs/1
  actuator/2 -> total flow sel/1
  veloc/1 -> actuator/3
  displ/1 -> actuator/2
  actuator/1 -> force/1
  cmd/1 -> actuator/1
  rtn press/1 -> actuator/5
  spl press/1 -> actuator/4

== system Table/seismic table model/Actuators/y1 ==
  note: Auxiliary diagnostic output vector: 1: valve opening 2: C1 pressure 3: C2 pressure 4: delta pressure 5: force 6: velocity 7: C1 flow 8: C2 flow 9: total flow 10: kinematic flow 11: compressibility flow 12: leakage flow
  note: Note: "1" and "2" denote actuator cylinders on either side of the actuator piston. With positive valve drive, oil is ported into cylinder 1, resulting in positive displacement.
  note: Parameter vector: 1: oil bulk modulus (force/displ^2) 2: servovalve natural frequency (Hz) 3: servovalve damping ratio 4: servovalve overlap 5: rated pressure (force/displ^2) 6: flow at rated pressure (displ^3/sec) 7: actuator piston area 1 (displ^2) 8: actuator piston area 2 (displ^2) 9: actuator usable stroke 1 (displ) 10: actuator usable stroke 2 (displ) 11: actuator end cushion length 1 (displ) 12: actuator end cushion length 2 (displ) 13: actuator parasitic damping factor 14: cross-chamber leakage factor (flow/press) 15: ratio port openings according to area 16: sample period (sec) Conversion factors used for converting signals from external (user) to internal (canonical) units: 17: displacement 18: velocity 19: force 20: pressure 21: flow
  cmd : Inport
  displ : Inport  Port=2
  veloc : Inport  Port=3
  spl press : Inport  Port=4
  rtn press : Inport  Port=5
  abs : Abs
  actuator : S-Function  FunctionName=actuator  Parameters=params
  total flow sel : Selector  Elements=9  InputPortWidth=12
  force : Outport
  flow : Outport  Port=2
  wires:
  spl press/1 -> actuator/4
  rtn press/1 -> actuator/5
  cmd/1 -> actuator/1
  actuator/1 -> force/1
  displ/1 -> actuator/2
  veloc/1 -> actuator/3
  actuator/2 -> total flow sel/1
  total flow sel/1 -> abs/1
  abs/1 -> flow/1

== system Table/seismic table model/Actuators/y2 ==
  note: Parameter vector: 1: oil bulk modulus (force/displ^2) 2: servovalve natural frequency (Hz) 3: servovalve damping ratio 4: servovalve overlap 5: rated pressure (force/displ^2) 6: flow at rated pressure (displ^3/sec) 7: actuator piston area 1 (displ^2) 8: actuator piston area 2 (displ^2) 9: actuator usable stroke 1 (displ) 10: actuator usable stroke 2 (displ) 11: actuator end cushion length 1 (displ) 12: actuator end cushion length 2 (displ) 13: actuator parasitic damping factor 14: cross-chamber leakage factor (flow/press) 15: ratio port openings according to area 16: sample period (sec) Conversion factors used for converting signals from external (user) to internal (canonical) units: 17: displacement 18: velocity 19: force 20: pressure 21: flow
  note: Note: "1" and "2" denote actuator cylinders on either side of the actuator piston. With positive valve drive, oil is ported into cylinder 1, resulting in positive displacement.
  note: Auxiliary diagnostic output vector: 1: valve opening 2: C1 pressure 3: C2 pressure 4: delta pressure 5: force 6: velocity 7: C1 flow 8: C2 flow 9: total flow 10: kinematic flow 11: compressibility flow 12: leakage flow
  cmd : Inport
  displ : Inport  Port=2
  veloc : Inport  Port=3
  spl press : Inport  Port=4
  rtn press : Inport  Port=5
  abs : Abs
  actuator : S-Function  FunctionName=actuator  Parameters=params
  total flow sel : Selector  Elements=9  InputPortWidth=12
  force : Outport
  flow : Outport  Port=2
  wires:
  abs/1 -> flow/1
  total flow sel/1 -> abs/1
  actuator/2 -> total flow sel/1
  veloc/1 -> actuator/3
  displ/1 -> actuator/2
  actuator/1 -> force/1
  cmd/1 -> actuator/1
  rtn press/1 -> actuator/5
  spl press/1 -> actuator/4

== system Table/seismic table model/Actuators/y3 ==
  note: Auxiliary diagnostic output vector: 1: valve opening 2: C1 pressure 3: C2 pressure 4: delta pressure 5: force 6: velocity 7: C1 flow 8: C2 flow 9: total flow 10: kinematic flow 11: compressibility flow 12: leakage flow
  note: Note: "1" and "2" denote actuator cylinders on either side of the actuator piston. With positive valve drive, oil is ported into cylinder 1, resulting in positive displacement.
  note: Parameter vector: 1: oil bulk modulus (force/displ^2) 2: servovalve natural frequency (Hz) 3: servovalve damping ratio 4: servovalve overlap 5: rated pressure (force/displ^2) 6: flow at rated pressure (displ^3/sec) 7: actuator piston area 1 (displ^2) 8: actuator piston area 2 (displ^2) 9: actuator usable stroke 1 (displ) 10: actuator usable stroke 2 (displ) 11: actuator end cushion length 1 (displ) 12: actuator end cushion length 2 (displ) 13: actuator parasitic damping factor 14: cross-chamber leakage factor (flow/press) 15: ratio port openings according to area 16: sample period (sec) Conversion factors used for converting signals from external (user) to internal (canonical) units: 17: displacement 18: velocity 19: force 20: pressure 21: flow
  cmd : Inport
  displ : Inport  Port=2
  veloc : Inport  Port=3
  spl press : Inport  Port=4
  rtn press : Inport  Port=5
  abs : Abs
  actuator : S-Function  FunctionName=actuator  Parameters=params
  total flow sel : Selector  Elements=9  InputPortWidth=12
  force : Outport
  flow : Outport  Port=2
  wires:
  spl press/1 -> actuator/4
  rtn press/1 -> actuator/5
  cmd/1 -> actuator/1
  actuator/1 -> force/1
  displ/1 -> actuator/2
  veloc/1 -> actuator/3
  actuator/2 -> total flow sel/1
  total flow sel/1 -> abs/1
  abs/1 -> flow/1

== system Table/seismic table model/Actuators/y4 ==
  note: Parameter vector: 1: oil bulk modulus (force/displ^2) 2: servovalve natural frequency (Hz) 3: servovalve damping ratio 4: servovalve overlap 5: rated pressure (force/displ^2) 6: flow at rated pressure (displ^3/sec) 7: actuator piston area 1 (displ^2) 8: actuator piston area 2 (displ^2) 9: actuator usable stroke 1 (displ) 10: actuator usable stroke 2 (displ) 11: actuator end cushion length 1 (displ) 12: actuator end cushion length 2 (displ) 13: actuator parasitic damping factor 14: cross-chamber leakage factor (flow/press) 15: ratio port openings according to area 16: sample period (sec) Conversion factors used for converting signals from external (user) to internal (canonical) units: 17: displacement 18: velocity 19: force 20: pressure 21: flow
  note: Note: "1" and "2" denote actuator cylinders on either side of the actuator piston. With positive valve drive, oil is ported into cylinder 1, resulting in positive displacement.
  note: Auxiliary diagnostic output vector: 1: valve opening 2: C1 pressure 3: C2 pressure 4: delta pressure 5: force 6: velocity 7: C1 flow 8: C2 flow 9: total flow 10: kinematic flow 11: compressibility flow 12: leakage flow
  cmd : Inport
  displ : Inport  Port=2
  veloc : Inport  Port=3
  spl press : Inport  Port=4
  rtn press : Inport  Port=5
  abs : Abs
  actuator : S-Function  FunctionName=actuator  Parameters=params
  total flow sel : Selector  Elements=9  InputPortWidth=12
  force : Outport
  flow : Outport  Port=2
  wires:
  abs/1 -> flow/1
  total flow sel/1 -> abs/1
  actuator/2 -> total flow sel/1
  veloc/1 -> actuator/3
  displ/1 -> actuator/2
  actuator/1 -> force/1
  cmd/1 -> actuator/1
  rtn press/1 -> actuator/5
  spl press/1 -> actuator/4

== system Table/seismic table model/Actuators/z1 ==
  note: Auxiliary diagnostic output vector: 1: valve opening 2: C1 pressure 3: C2 pressure 4: delta pressure 5: force 6: velocity 7: C1 flow 8: C2 flow 9: total flow 10: kinematic flow 11: compressibility flow 12: leakage flow
  note: Note: "1" and "2" denote actuator cylinders on either side of the actuator piston. With positive valve drive, oil is ported into cylinder 1, resulting in positive displacement.
  note: Parameter vector: 1: oil bulk modulus (force/displ^2) 2: servovalve natural frequency (Hz) 3: servovalve damping ratio 4: servovalve overlap 5: rated pressure (force/displ^2) 6: flow at rated pressure (displ^3/sec) 7: actuator piston area 1 (displ^2) 8: actuator piston area 2 (displ^2) 9: actuator usable stroke 1 (displ) 10: actuator usable stroke 2 (displ) 11: actuator end cushion length 1 (displ) 12: actuator end cushion length 2 (displ) 13: actuator parasitic damping factor 14: cross-chamber leakage factor (flow/press) 15: ratio port openings according to area 16: sample period (sec) Conversion factors used for converting signals from external (user) to internal (canonical) units: 17: displacement 18: velocity 19: force 20: pressure 21: flow
  cmd : Inport
  displ : Inport  Port=2
  veloc : Inport  Port=3
  spl press : Inport  Port=4
  rtn press : Inport  Port=5
  abs : Abs
  actuator : S-Function  FunctionName=actuator  Parameters=params
  total flow sel : Selector  Elements=9  InputPortWidth=12
  force : Outport
  flow : Outport  Port=2
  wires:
  spl press/1 -> actuator/4
  rtn press/1 -> actuator/5
  cmd/1 -> actuator/1
  actuator/1 -> force/1
  displ/1 -> actuator/2
  veloc/1 -> actuator/3
  actuator/2 -> total flow sel/1
  total flow sel/1 -> abs/1
  abs/1 -> flow/1

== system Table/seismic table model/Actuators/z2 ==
  note: Parameter vector: 1: oil bulk modulus (force/displ^2) 2: servovalve natural frequency (Hz) 3: servovalve damping ratio 4: servovalve overlap 5: rated pressure (force/displ^2) 6: flow at rated pressure (displ^3/sec) 7: actuator piston area 1 (displ^2) 8: actuator piston area 2 (displ^2) 9: actuator usable stroke 1 (displ) 10: actuator usable stroke 2 (displ) 11: actuator end cushion length 1 (displ) 12: actuator end cushion length 2 (displ) 13: actuator parasitic damping factor 14: cross-chamber leakage factor (flow/press) 15: ratio port openings according to area 16: sample period (sec) Conversion factors used for converting signals from external (user) to internal (canonical) units: 17: displacement 18: velocity 19: force 20: pressure 21: flow
  note: Note: "1" and "2" denote actuator cylinders on either side of the actuator piston. With positive valve drive, oil is ported into cylinder 1, resulting in positive displacement.
  note: Auxiliary diagnostic output vector: 1: valve opening 2: C1 pressure 3: C2 pressure 4: delta pressure 5: force 6: velocity 7: C1 flow 8: C2 flow 9: total flow 10: kinematic flow 11: compressibility flow 12: leakage flow
  cmd : Inport
  displ : Inport  Port=2
  veloc : Inport  Port=3
  spl press : Inport  Port=4
  rtn press : Inport  Port=5
  abs : Abs
  actuator : S-Function  FunctionName=actuator  Parameters=params
  total flow sel : Selector  Elements=9  InputPortWidth=12
  force : Outport
  flow : Outport  Port=2
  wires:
  abs/1 -> flow/1
  total flow sel/1 -> abs/1
  actuator/2 -> total flow sel/1
  veloc/1 -> actuator/3
  displ/1 -> actuator/2
  actuator/1 -> force/1
  cmd/1 -> actuator/1
  rtn press/1 -> actuator/5
  spl press/1 -> actuator/4

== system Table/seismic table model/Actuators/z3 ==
  note: Auxiliary diagnostic output vector: 1: valve opening 2: C1 pressure 3: C2 pressure 4: delta pressure 5: force 6: velocity 7: C1 flow 8: C2 flow 9: total flow 10: kinematic flow 11: compressibility flow 12: leakage flow
  note: Note: "1" and "2" denote actuator cylinders on either side of the actuator piston. With positive valve drive, oil is ported into cylinder 1, resulting in positive displacement.
  note: Parameter vector: 1: oil bulk modulus (force/displ^2) 2: servovalve natural frequency (Hz) 3: servovalve damping ratio 4: servovalve overlap 5: rated pressure (force/displ^2) 6: flow at rated pressure (displ^3/sec) 7: actuator piston area 1 (displ^2) 8: actuator piston area 2 (displ^2) 9: actuator usable stroke 1 (displ) 10: actuator usable stroke 2 (displ) 11: actuator end cushion length 1 (displ) 12: actuator end cushion length 2 (displ) 13: actuator parasitic damping factor 14: cross-chamber leakage factor (flow/press) 15: ratio port openings according to area 16: sample period (sec) Conversion factors used for converting signals from external (user) to internal (canonical) units: 17: displacement 18: velocity 19: force 20: pressure 21: flow
  cmd : Inport
  displ : Inport  Port=2
  veloc : Inport  Port=3
  spl press : Inport  Port=4
  rtn press : Inport  Port=5
  abs : Abs
  actuator : S-Function  FunctionName=actuator  Parameters=params
  total flow sel : Selector  Elements=9  InputPortWidth=12
  force : Outport
  flow : Outport  Port=2
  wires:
  spl press/1 -> actuator/4
  rtn press/1 -> actuator/5
  cmd/1 -> actuator/1
  actuator/1 -> force/1
  displ/1 -> actuator/2
  veloc/1 -> actuator/3
  actuator/2 -> total flow sel/1
  total flow sel/1 -> abs/1
  abs/1 -> flow/1

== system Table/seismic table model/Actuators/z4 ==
  note: Parameter vector: 1: oil bulk modulus (force/displ^2) 2: servovalve natural frequency (Hz) 3: servovalve damping ratio 4: servovalve overlap 5: rated pressure (force/displ^2) 6: flow at rated pressure (displ^3/sec) 7: actuator piston area 1 (displ^2) 8: actuator piston area 2 (displ^2) 9: actuator usable stroke 1 (displ) 10: actuator usable stroke 2 (displ) 11: actuator end cushion length 1 (displ) 12: actuator end cushion length 2 (displ) 13: actuator parasitic damping factor 14: cross-chamber leakage factor (flow/press) 15: ratio port openings according to area 16: sample period (sec) Conversion factors used for converting signals from external (user) to internal (canonical) units: 17: displacement 18: velocity 19: force 20: pressure 21: flow
  note: Note: "1" and "2" denote actuator cylinders on either side of the actuator piston. With positive valve drive, oil is ported into cylinder 1, resulting in positive displacement.
  note: Auxiliary diagnostic output vector: 1: valve opening 2: C1 pressure 3: C2 pressure 4: delta pressure 5: force 6: velocity 7: C1 flow 8: C2 flow 9: total flow 10: kinematic flow 11: compressibility flow 12: leakage flow
  cmd : Inport
  displ : Inport  Port=2
  veloc : Inport  Port=3
  spl press : Inport  Port=4
  rtn press : Inport  Port=5
  abs : Abs
  actuator : S-Function  FunctionName=actuator  Parameters=params
  total flow sel : Selector  Elements=9  InputPortWidth=12
  force : Outport
  flow : Outport  Port=2
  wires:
  abs/1 -> flow/1
  total flow sel/1 -> abs/1
  actuator/2 -> total flow sel/1
  veloc/1 -> actuator/3
  displ/1 -> actuator/2
  actuator/1 -> force/1
  cmd/1 -> actuator/1
  rtn press/1 -> actuator/5
  spl press/1 -> actuator/4

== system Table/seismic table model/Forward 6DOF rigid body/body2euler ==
  rpw : Inport
  11 : Fcn  Expr=cos(u[2])
  12 : Fcn  Expr=0
  13 : Fcn  Expr=-sin(u[2])
  21 : Fcn  Expr=sin(u[2])*tan(u[1])
  22 : Fcn  Expr=1
  23 : Fcn  Expr=cos(u[2])*tan(u[1])
  31 : Fcn  Expr=sin(u[2])/cos(u[1])
  32 : Fcn  Expr=0
  33 : Fcn  Expr=cos(u[2])/cos(u[1])
  9x1->3x3 : simulink/Math Operations/Reshape  OutputDimensionality=Customize  OutputDimensions=[3,3]
  Mux2 : Mux  Orientation=down  Inputs=9
  out : Outport
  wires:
  9x1->3x3/1 -> out/1
  11/1 -> Mux2/1
  21/1 -> Mux2/2
  31/1 -> Mux2/3
  rpw/1 -> 31/1, 21/1, 11/1, 32/1, 22/1, 12/1, 33/1, 23/1, 13/1
  12/1 -> Mux2/4
  22/1 -> Mux2/5
  32/1 -> Mux2/6
  Mux2/1 -> 9x1->3x3/1
  13/1 -> Mux2/7
  23/1 -> Mux2/8
  33/1 -> Mux2/9

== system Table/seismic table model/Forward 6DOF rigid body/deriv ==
  inp : Inport
  1/T : Gain  Gain=1/T
  Sum : Sum  Inputs=|+-
  Unit Delay : UnitDelay  SampleTime=-1
  out : Outport
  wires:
  inp/1 -> Sum/1, Unit Delay/1
  Unit Delay/1 -> Sum/2
  Sum/1 -> 1/T/1
  1/T/1 -> out/1

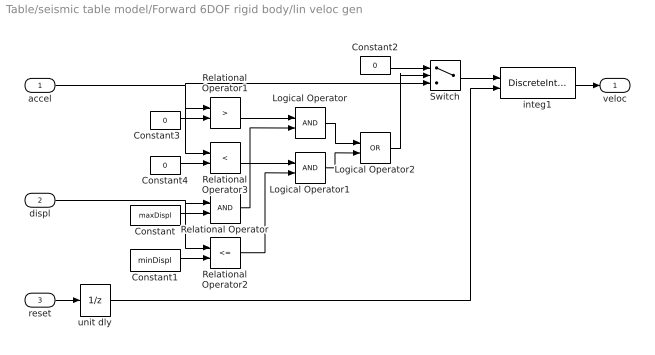
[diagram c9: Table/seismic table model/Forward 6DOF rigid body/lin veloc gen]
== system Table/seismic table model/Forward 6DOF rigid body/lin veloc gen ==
  accel : Inport
  displ : Inport  Port=2
  reset : Inport  Port=3
  Constant : Constant  Value=maxDispl
  Constant1 : Constant  Value=minDispl
  Constant2 : Constant  Value=0
  Constant3 : Constant  Value=0
  Constant4 : Constant  Value=0
  Logical Operator : Logic
  Logical Operator1 : Logic
  Logical Operator2 : Logic  Operator=OR
  Relational Operator : RelationalOperator
  Relational Operator1 : RelationalOperator  Operator=>
  Relational Operator2 : RelationalOperator  Operator=<=
  Relational Operator3 : RelationalOperator  Operator=<
  Switch : Switch  Threshold=0.5
  integ1 : DiscreteIntegrator  ExternalReset=either  LimitOutput=on  UpperSaturationLimit=maxVeloc  LowerSaturationLimit=minVeloc  SampleTime=-1
  unit dly : UnitDelay  SampleTime=-1
  veloc : Outport
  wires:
  integ1/1 -> veloc/1
  Constant/1 -> Relational Operator/2
  Relational Operator/1 -> Logical Operator/2
  Relational Operator2/1 -> Logical Operator1/2
  Constant1/1 -> Relational Operator2/2
  accel/1 -> Relational Operator3/1, Relational Operator1/1, Switch/3
  Constant3/1 -> Relational Operator1/2
  Relational Operator1/1 -> Logical Operator/1
  Constant4/1 -> Relational Operator3/2
  Relational Operator3/1 -> Logical Operator1/1
  Logical Operator/1 -> Logical Operator2/1
  Constant2/1 -> Switch/1
  Logical Operator2/1 -> Switch/2
  Switch/1 -> integ1/1
  unit dly/1 -> integ1/2
  Logical Operator1/1 -> Logical Operator2/2
  displ/1 -> Relational Operator/1, Relational Operator2/1
  reset/1 -> unit dly/1
